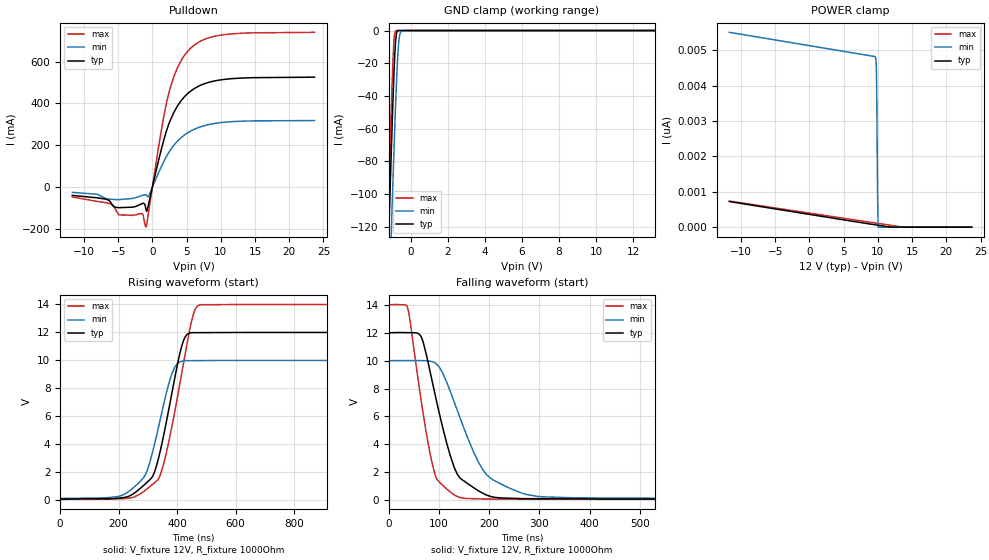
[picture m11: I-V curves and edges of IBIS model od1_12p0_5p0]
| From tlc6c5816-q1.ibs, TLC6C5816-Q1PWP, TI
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|   od1_12p0_5p0 Model
[Model]   od1_12p0_5p0
Model_type   Open_drain
Polarity   Inverting
Vmeas = 6
Vref = 12
Cref = 2pF
Rref = 1000
|   typ   min   max
C_comp   3.695pF   3.324pF   3.764pF
| Where Nom  PVT is Nominal Process, 12.0V, 27C
|   Fast PVT is Strong Process,  14.0V, -40C
|   Slow PVT is Weak Process,   10.0V, 150C
[Voltage Range]   12   10   14
|Junction Temperature
[Temperature Range]   27   150   -40
[Pullup Reference]   12   10   14
[Pulldown Reference]   0   -0   0
[Power Clamp Reference]   12   10   14
[GND Clamp Reference]   0   0   0
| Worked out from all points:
|   slope of the pulldown table from 0 to 1.8 V, typ, clamps not added: 7.52 ohm
|   GND clamp passes 1 mA (typ) near -0.76 V on its own axis
|   falling waveform, V_fixture 12V, R_fixture 1000Ohm: 20-80 % time 49.5ns typ, 69.1ns min, 36.6ns max; typ from 12 V to 0.082 V
|   rising waveform, V_fixture 12V, R_fixture 1000Ohm: 20-80 % time 70.8ns typ, 70.7ns min, 77.2ns max; typ from 0.082 V to 12 V
[Pulldown]
|   Voltage   I(typ)   I(min)   I(max)
-11.7V    -38.64mA   -24.27mA   -46.16mA
-6.142V   -69.34mA   -57.11mA   -78.58mA
-4.903V   -97.36mA   -59.03mA   -131.4mA
-1.469V   -77.4mA    -38.88mA   -126mA
-903mV    -109.6mA   -36.74mA   -190.3mA
-549mV    -80.17mA   -43.53mA   -118.5mA
1.15V     160.1mA    86.61mA    239.8mA
2.141V    276.3mA    151.1mA    412.7mA
3.593V    383.6mA    217.6mA    564.6mA
5.15V     446.7mA    259.7mA    648.5mA
10.07V    512.9mA    308.8mA    726.6mA
23.7V     525.4mA    318.4mA    739.5mA
[GND Clamp]
|   Voltage   I(typ)   I(min)   I(max)
-11.7V    -5.142A    -4.912A    -5.294A
-1.257V   -147.7mA   -196.2mA   -122.2mA
-1.115V   -94.13mA   -143.7mA   -67.68mA
-1.045V   -68.45mA   -118.2mA   -42.16mA
-973.8mV  -44.18mA   -93.26mA   -19.47mA
-903mV    -22.64mA   -69.32mA   -4.129mA
-832.2mV  -7.051mA   -46.92mA   -263.1uA
-796.8mV  -2.903mA   -36.59mA   -56.31uA
-690.6mV  -89.96uA   -11.86mA   -687nA
-619.8mV  -7.619uA   -3.44mA    -55.01nA
-336.6mV  -444.4pA   -3.796uA   -12.88pA
23.7V     0A         0A         0A
[POWER Clamp]
|   Voltage   I(typ)   I(min)   I(max)
-11.7V    723.7pA    5.506nA    737.5pA
9.611V    65.75pA    4.814nA    118.3pA
9.717V    62.54pA    4.73nA     115.2pA
9.752V    61.47pA    4.619nA    114.2pA
9.788V    60.39pA    4.382nA    113.2pA
9.823V    59.32pA    3.921nA    112.1pA
9.859V    58.25pA    3.178nA    111.1pA
9.929V    56.11pA    1.456nA    109.1pA
9.965V    55.05pA    778.7pA    108.1pA
10.04V    52.91pA    0A         106pA
13.96V    0A         0A         455fA
23.7V     0A         0A         0A
[Ramp]
R_load = 1000
|   typ   min   max
dV/dt_r   7.15068/7.08186e-08   5.92493/7.07317e-08   8.36119/7.72008e-08
dV/dt_f   7.15071/4.94807e-08   5.92497/6.90541e-08   8.36121/3.66076e-08
[Falling Waveform]
V_fixture = 12V
V_fixture_min = 10V
V_fixture_max = 14V
R_fixture = 1000Ohm
C_fixture = 0F
|   Time   V(typ)   V(min)   V(max)
0s        12V        10V        14V
37.79ns   12.01V     10.01V     13.76V
64.36ns   11.73V     10V        7.203V
81.08ns   9.437V     9.965V     3.589V
95.94ns   6.997V     9.733V     1.507V
123.6ns   3.081V     7.703V     568.7mV
147.6ns   1.435V     5.382V     151.5mV
195.5ns   363.7mV    1.811V     84.33mV
308ns     108.1mV    240.7mV    71.01mV
2.5us     82.15mV    125mV      64.65mV
[Rising Waveform]
V_fixture = 12V
V_fixture_min = 10V
V_fixture_max = 14V
R_fixture = 1000Ohm
C_fixture = 0F
|   Time   V(typ)   V(min)   V(max)
0s        82.15mV    125mV      64.65mV
230.5ns   253.1mV    564.9mV    140.5mV
291ns     1.16V      1.809V     712.2mV
317.6ns   1.759V     3.557V     1.16V
333.6ns   2.771V     4.969V     1.443V
378.2ns   7.216V     8.793V     4.849V
416.9ns   11.1V      9.939V     9.193V
454ns     11.99V     9.984V     13.17V
477.4ns   11.99V     9.987V     13.97V
2.5us     12V        10V        14V
